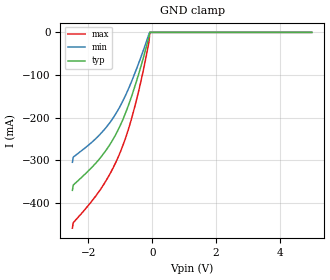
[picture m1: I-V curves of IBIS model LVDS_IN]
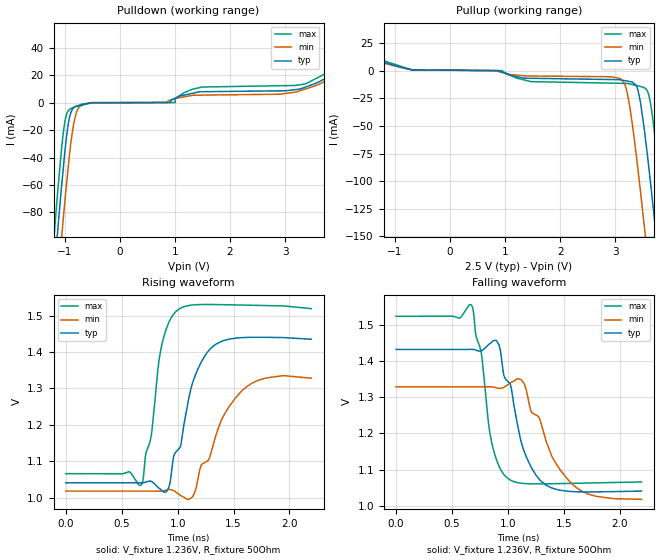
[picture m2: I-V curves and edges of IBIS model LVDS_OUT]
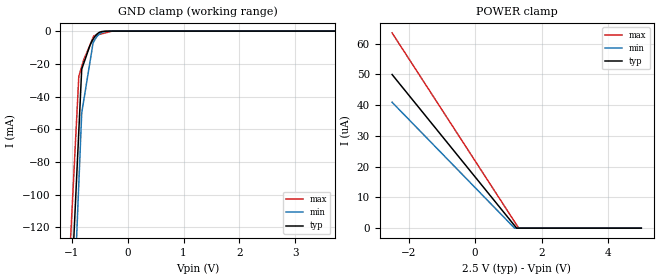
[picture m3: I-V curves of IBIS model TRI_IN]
| Texas Instruments Incorporated
| 2:8 Low Additive Jitter LVDS buffer
| Marketing part#   Voltage Range   Package-type   #pins/pkg drawing
| CDCLVD1208   2.375V-3.625V   QFN   28-pin QFN
[IBIS Ver]   4.0
[File name]   cdclvd1208.ibs
[File Rev]   1.2
[Date]   10/23/2018
[Source]   spectre simulations
   Texas Instruments Incorporated.
   Analog eLab Design Center, HPA
   12500 TI Blvd
   Dallas, TX -75243
   For Support e-mail: elab_scm_ibis@list.ti.com
[Notes]   Revision History:
   Rev 1.2: 10/23/2018
   - TRI_IN model updated to reflect true electrical behavior.
   - VBB_OUT model removed  due  to inaccurary in describing
   termination behavior.
   Rev 1.1: 8/29/2013
   - Updated LVDS_IN to correct POWER and GROUND Clamp models.
   Rev 1.0: 07/06/2010
   - C_comp although listed in numberical order of value are obtained from varying PVT conditions.
   For PVT conditions for eachspecific value, refer to the buffer description under repective [Model].
   IBIS model user is responsible for using appropriate C_comp to simulate for Signal Integrity.
   - TISPice simulation of Clamp current does not match silicon
   - POWER and GND clamp for TRI_IN, D_REB_IN non-monotonic due circuit design
   - GND clamp for LVDS_IN non-monotonic due to circuit design
   - LVDS_OUT pullup/pulldown non-monotonic as a result of circuit design
[Disclaimer] This model is designed as an aid for customers of Texas Instruments.
 TI and its licensors and suppliers make no warranties, either expressed
 or implied, with respect to this  model, including the warranties of
 merchantability or fitness for a particular purpose.
 The model is provided solely on an "as is" basis. The entire risk as to
 its quality and performance is with the customer.
[Copyright] (C)Copyright 2013 Texas Instruments Incorporated.
   All rights reserved.
|   Component CDCLVD1208
[Component]   CDCLVD1208
[Manufacturer]  Texas Instruments Incorporated
[Package]   |QFN (RHD) 28-pin
|   typ   min   max
R_pkg   0.1218   0.05022   0.15010
L_pkg   1.7704nH   1.61819nH   2.20538nH
C_pkg   0.16629pF   0.15643pF   0.24429pF
[Pin]   signal_name   model_name   R_pin   L_pin   C_pin
1   GND   GND   0.07422  1.74079n  0.22060p
2   OUTP7   LVDS_OUT   0.13406  1.90082n  0.17398p
3   OUTN7   LVDS_OUT   0.12451  1.75134n  0.16133p
4   IN_SEL   TRI_IN   0.12065  1.69116n  0.15677p
5   INP1   LVDS_IN   0.12310  1.72944n  0.15959p
6   INN1   LVDS_IN   0.13146  1.86023n  0.16888p
7   VAC_REF1   NC   0.14660  2.10008n  0.17055p
8   VCC   POWER   0.05022  1.72325n  0.24429p
9   INP0   LVDS_IN   0.13687  1.94322n  0.17789p
10   INN0   LVDS_IN   0.12620  1.77474n  0.16323p
11   VAC_REF0   NC   0.12097  1.69186n  0.15704p
12   OUTP0   LVDS_OUT   0.12199  1.70664n  0.15829p
13   OUTN0   LVDS_OUT   0.12910  1.81703n  0.16785p
14   GND   GND   0.07281  1.61819n  0.22369p
15   VCC   POWER   0.15010  2.14718n  0.17752p
16   OUTP1   LVDS_OUT   0.13406  1.89222n  0.17202p
17   OUTN1   LVDS_OUT   0.12451  1.74204n  0.16097p
18   OUTP2   LVDS_OUT   0.12065  1.68156n  0.15643p
19   OUTN2   LVDS_OUT   0.12310  1.72004n  0.15921p
20   OUTP3   LVDS_OUT   0.13146  1.85151n  0.16830p
21   OUTN3   LVDS_OUT   0.14660  2.09208n  0.16760p
22   OUTP4   LVDS_OUT   0.15376  2.20538n  0.17530p
23   OUTN4   LVDS_OUT   0.13688  1.93813n  0.17483p
24   OUTP5   LVDS_OUT   0.12621  1.77175n  0.16296p
25   OUTN5   LVDS_OUT   0.12098  1.69126n  0.15699p
26   OUTP6   LVDS_OUT   0.12201  1.70855n  0.15826p
27   OUTN6   LVDS_OUT   0.12912  1.82123n  0.16629p
28   VCC   POWER   0.14328  2.04688n  0.16834p
[Diff_pin]   inv_pin   vdiff   tdelay_typ   tdelay_min   tdelay_max
| The 'OUTPx' pin is Diff_pin and the 'OUTNx' pin is the inv_pin
| The 'INPx' pin is Diff_pin and the 'INNx' pin is the inv_pin
2   3   0.200   0 0 0
5   6   0.200   0 0 0
9   10   0.200   0 0 0
12   13   0.200   0 0 0
16   17   0.200   0 0 0
18   19   0.200   0 0 0
20   21   0.200   0 0 0
22   23   0.200   0 0 0
24   25   0.200   0 0 0
26   27   0.200   0 0 0
| Models and submodels in the file (3): LVDS_IN (Input), LVDS_OUT (Output), TRI_IN (Input)
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|   LVDS_IN Input Model
[Model]   LVDS_IN
Model_type   Input
|Signals   INN0,INP0,INN1,INP1
Vinh = 1.6
Vinl = 0.3
| variable   typ   min   max
|   (nom PVT)   (slow PVT)   (fast PVT)
C_comp   3.121pF   2.849pF   3.193pF
| Ccomp comes from PVT, calculated at 800MHz.
| Nom PVT is nom process, 2.5V, 25C
| slow PVT is weak process, 2.375V, 105C
| Fast process is strong process, 2.625V, -40C
|   typ   min   max
[Voltage Range]   2.5   2.375   2.625
[Temperature Range]   25   105   -40
[Power Clamp Reference]   2.5   2.375   2.625
[GND Clamp Reference]   0   0   0
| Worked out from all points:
|   GND clamp passes 1 mA (typ) near -0.08 V on its own axis
[GND Clamp]
|   Voltage   I(typ)   I(min)   I(max)
-2.5V     -370.8mA   -304.9mA   -459.4mA
-2.475V   -358.5mA   -293mA     -446.8mA
-1.9V     -317.5mA   -258.4mA   -396.7mA
-1.5V     -282.1mA   -228.1mA   -354.5mA
-1.225V   -250.8mA   -200.9mA   -318mA
-975mV    -214.1mA   -169mA     -276.3mA
-700mV    -161.8mA   -124.9mA   -216.1mA
-450mV    -104.2mA   -77.57mA   -145.7mA
-150mV    -24.38mA   -14.67mA   -41.36mA
-100mV    -9.871mA   -3.55mA    -21.64mA
-75.01mV  0A         0A         0A
5V        0A         0A         0A
[POWER Clamp]
|   Voltage   I(typ)   I(min)   I(max)
-2.5V     0A         0A         0A
-2.475V   0A         0A         0A
-2.45V    0A         0A         0A
5V        0A         0A         0A
|   LVDS_OUT Model
[Model]   LVDS_OUT
Model_type   Output
| Signals   OUTP0,OUTN0,OUTP1,OUTN1,OUTP2,OUTN2,OUTP3,OUTN3,OUTP4,OUTN4,OUTP5,OUTN5,OUTP6,OUTN6,OUTP7,OUTN7
Polarity   Non-Inverting
Vmeas = 1.25
Vref = 1.25
Cref = 15pF
Rref = 50
| variable   typ   min   max
|   (nom PVT)   (slow PVT)   (fast PVT)
C_comp   1.275pF   1.175pF   1.317pF
| Ccomp comes from PVT corner simulations
| Nom PVT is nom process, 2.5V, 25C
| slow PVT is weak process, 2.375V, 105C
| Fast process is strong process, 2.625V, -40C
[Voltage Range]   2.5   2.375   2.625
[Temperature Range]   25   105   -40
[Pullup Reference]   2.5   2.375   2.625
[Pulldown Reference]   0   0   0
[Power Clamp Reference]   2.5   2.375   2.625
[GND Clamp Reference]   0   0   0
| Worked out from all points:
|   slope of the pulldown table from 0 to 0.375 V, typ, clamps not added: 11.9 kohm
|   slope of the pullup table from 0 to 0.375 V, typ, clamps not added: 2.06 kohm
|   falling waveform, V_fixture 1.236V, R_fixture 50Ohm: 20-80 % time 216ps typ, 313ps min, 114ps max; typ from 1.43 V to 1.04 V
|   rising waveform, V_fixture 1.236V, R_fixture 50Ohm: 20-80 % time 213ps typ, 297ps min, 111ps max; typ from 1.04 V to 1.44 V
[Pulldown]
|   Voltage   I(typ)   I(min)   I(max)
-2.5V     -819.9mA   -841.2mA   -808.9mA
-1.205V   -132.7mA   -170.8mA   -104.8mA
-1.179V   -119.9mA   -157.8mA   -91.4mA
-1.126V   -94.38mA   -132.6mA   -65.81mA
-1.057V   -62.54mA   -100.1mA   -34.83mA
-992.5mV  -35.05mA   -71.07mA   -13.52mA
-904.2mV  -9.792mA   -35.76mA   -4.869mA
-801.5mV  -2.839mA   -9.874mA   -2.967mA
-497.6mV  -107.4uA   -219.6uA   -77.81uA
1.006V    3.123mA    2.958mA    13.07uA
3.348V    10.9mA     9.549mA    13.39mA
4.992V    48.76mA    47.89mA    54.44mA
[Pullup]
|   Voltage   I(typ)   I(min)   I(max)
-2.5V     34.99mA    35.32mA    37.69mA
-673.6mV  752.9uA    742.8uA    631.1uA
3.09V     -8.286mA   -7.075mA   -11.46mA
3.202V    -9.311mA   -16.77mA   -11.57mA
3.31V     -10.29mA   -48.27mA   -12.56mA
3.416V    -18.21mA   -90.66mA   -13.83mA
3.525V    -51.64mA   -139.2mA   -15.42mA
3.637V    -99.27mA   -190.6mA   -28.34mA
3.71V     -133.1mA   -225.4mA   -54.42mA
3.766V    -159.3mA   -252.7mA   -79.01mA
3.928V    -237.8mA   -331.5mA   -155.2mA
4.992V    -776.9mA   -866.8mA   -698.2mA
[Ramp]
R_load = 50
|   typ   min   max
dV/dt_r   0.238696/2.15967e-10   0.19168/3.14155e-10   0.275901/1.13765e-10
dV/dt_f   0.234348/2.15967e-10   0.186163/3.14155e-10   0.274079/1.13765e-10
[Falling Waveform]
V_fixture = 1.236V
V_fixture_min = 1.173V
V_fixture_max = 1.294V
R_fixture = 50Ohm
C_fixture = 0F
|   Time   V(typ)   V(min)   V(max)
0s        1.431V     1.328V     1.523V
675ps     1.432V     1.328V     1.553V
765ps     1.428V     1.328V     1.417V
855ps     1.451V     1.328V     1.176V
920ps     1.445V     1.324V     1.11V
1.01ns    1.34V      1.337V     1.073V
1.135ns   1.16V      1.342V     1.062V
1.305ns   1.066V     1.219V     1.061V
1.62ns    1.039V     1.049V     1.062V
2.195ns   1.041V     1.018V     1.066V
[Rising Waveform]
V_fixture = 1.236V
V_fixture_min = 1.173V
V_fixture_max = 1.294V
R_fixture = 50Ohm
C_fixture = 0F
|   Time   V(typ)   V(min)   V(max)
0s        1.041V     1.018V     1.066V
675ps     1.04V      1.018V     1.035V
765ps     1.044V     1.018V     1.172V
855ps     1.021V     1.018V     1.415V
920ps     1.027V     1.022V     1.481V
1.01ns    1.133V     1.009V     1.518V
1.135ns   1.317V     1.004V     1.53V
1.305ns   1.413V     1.13V      1.531V
1.62ns    1.44V      1.306V     1.529V
2.195ns   1.435V     1.328V     1.52V
|   TRI_IN Input Model
[Model]   TRI_IN
Model_type   Input
Vinl = 0.475
Vinh = 1.8375
|   typ   min   max
C_comp   1.974pF   1.947pF   1.983pF
[Voltage Range]   2.5   2.375   2.625
[Temperature Range]   25   105   -40
[Power Clamp Reference]   2.5   2.375   2.625
[GND Clamp Reference]   0   0   0
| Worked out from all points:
|   GND clamp passes 1 mA (typ) near -0.51 V on its own axis
[GND Clamp]
|   Voltage   I(typ)   I(min)   I(max)
-2.5V     -1.519A    -1.599A    -1.46A
-1.383V   -435.2mA   -519.8mA   -372mA
-872mV    -61.4mA    -93.54mA   -27.86mA
-820mV    -23.3mA    -50.1mA    -21.6mA
-782.5mV  -19.62mA   -42.18mA   -17.41mA
-670mV    -8.564mA   -18.42mA   -8.334mA
-617.5mV  -5.055mA   -7.338mA   -4.098mA
-602.5mV  -4.217mA   -6.329mA   -2.888mA
-497.5mV  -686.1uA   -1.614mA   -1.968mA
-415mV    -96.99uA   -336uA     -1.246mA
-275.7mV  -21.08uA   -26.56uA   -26.45uA
5V        0A         0A         0A
[POWER Clamp]
|   Voltage   I(typ)   I(min)   I(max)
-2.5V     49.93uA    40.92uA    63.45uA
1.183V    882.3nA    41.92nA    2.147uA
1.242V    83.42nA    0A         1.149uA
1.31V     0A         0A         25.11nA
5V        0A         0A         0A
